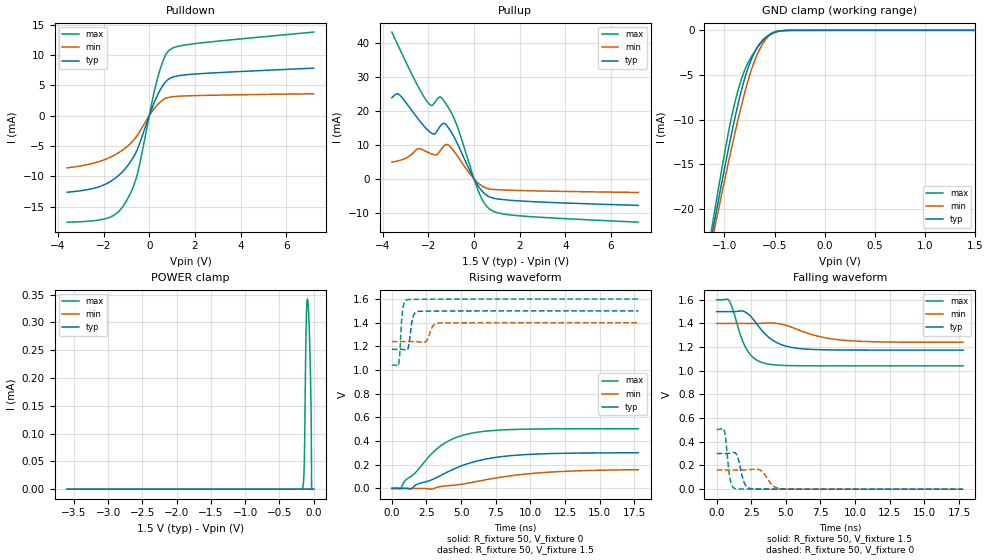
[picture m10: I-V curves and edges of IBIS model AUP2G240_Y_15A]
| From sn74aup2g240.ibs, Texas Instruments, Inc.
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[Model]   AUP2G240_Y_15A
Model_type  3-state
Enable   Active-Low
Vref =   0
Rref =   1E6
Cref =   30p
Vmeas =   0.75
| variable   typ   min   max
C_comp   2.15pF   1.95pF   2.46pF
| C_pullup   2.93pF   2.16pF   3.64pF
| C_pulldown   2.53pF   2.25pF   2.88pF
| C_tri-state   2.15pF   1.95pF   2.46pF
[Temperature Range]   40   100   -40
| Ambient temperature   25   85   -40
[Voltage range]   1.5   1.4   1.6
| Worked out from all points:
|   slope of the pulldown table from 0 to 0.225 V, typ, clamps not added: 101 ohm
|   slope of the pullup table from 0 to 0.225 V, typ, clamps not added: 90.7 ohm
|   GND clamp passes 1 mA (typ) near -0.61 V on its own axis
|   rising waveform, R_fixture 50, V_fixture 0: 20-80 % time 3.92ns typ, 5.36ns min, 2.76ns max; typ from 0 V to 0.301 V
|   falling waveform, R_fixture 50, V_fixture 1.5: 20-80 % time 1.67ns typ, 2.73ns min, 1.07ns max; typ from 1.5 V to 1.18 V
|   rising waveform, R_fixture 50, V_fixture 1.5: 20-80 % time 232ps typ, 317ps min, 180ps max; typ from 1.18 V to 1.5 V
|   falling waveform, R_fixture 50, V_fixture 0: 20-80 % time 381ps typ, 592ps min, 272ps max; typ from 0.302 V to 0 V
[GND Clamp]
| AUP2G240_Y_15A
|   Voltage   I(typ)   I(min)   I(max)
-3.6V     -191.7mA   -177.9mA   -208.5mA
-1.13V    -23.31mA   -24.02mA   -22.49mA
-1.105V   -21.79mA   -22.63mA   -20.79mA
-1.085V   -20.58mA   -21.53mA   -19.44mA
-950mV    -12.76mA   -14.3mA    -10.91mA
-850mV    -7.621mA   -9.344mA   -6.192mA
-785mV    -4.955mA   -6.469mA   -4.124mA
-720mV    -2.969mA   -4.074mA   -2.762mA
-650mV    -1.522mA   -2.167mA   -1.616mA
-580mV    -733.4uA   -902.1uA   -734uA
-390mV    -21.99uA   -24.65uA   -8.299uA
1.5V      139.3pA    22.28nA    27.28pA
[POWER Clamp]
| AUP2G240_Y_15A
|   Voltage   I(typ)   I(min)   I(max)
-3.6V     1.555nA    3.017nA    543.3pA
-170mV    947.8pA    3.23nA     623.5nA
-140mV    6.153nA    7.576nA    33.92uA
-130mV    14.96nA    10.7nA     97.54uA
-110mV    84.92nA    19.18nA    292.2uA
-100mV    170.9nA    22.28nA    332.3uA
-90mV     274.7nA    22.96nA    342.1uA
-70mV     286.4nA    16.34nA    307.8uA
-45mV     32.5nA     4.747nA    195.4uA
-35mV     468.4pA    2.585nA    123.1uA
-30mV     327.7pA    1.919nA    35.79pA
0V        0A         0A         0A
[Pulldown]
| AUP2G240_Y_15A
|   Voltage   I(typ)   I(min)   I(max)
-3.6V     -12.62mA   -8.605mA   -17.56mA
-1.79V    -11.04mA   -6.985mA   -16.83mA
-1.38V    -9.961mA   -6.191mA   -15.93mA
-1.02V    -8.588mA   -5.241mA   -14.16mA
-725mV    -7.016mA   -4.193mA   -11.94mA
-525mV    -5.567mA   -3.252mA   -9.657mA
150mV     1.53mA     832.4uA    2.806mA
420mV     3.835mA    2.043mA    6.955mA
670mV     5.357mA    2.767mA    9.628mA
900mV     6.139mA    3.055mA    10.86mA
1.995V    6.857mA    3.303mA    11.87mA
7.2V      7.827mA    3.609mA    13.77mA
[Pullup]
| AUP2G240_Y_15A
|   Voltage   I(typ)   I(min)   I(max)
-3.6V     23.95mA    4.976mA    43.35mA
-3.25V    24.72mA    5.488mA    38.28mA
-2.46V    17.83mA    8.92mA     27.43mA
-2.06V    14.65mA    7.989mA    22.9mA
-1.74V    13.25mA    7.129mA    22.39mA
-1.475V   15.6mA     8.413mA    24.19mA
-1.17V    15.57mA    10.16mA    21.56mA
-730mV    10.45mA    6.821mA    15.42mA
200mV     -2.247mA   -1.333mA   -3.769mA
690mV     -5.334mA   -2.972mA   -8.934mA
1.94V     -6.46mA    -3.399mA   -10.85mA
7.2V      -7.803mA   -3.988mA   -12.76mA
[Ramp]
| AUP2G240_Y_15A
| variable   typ   min   max
dV/dt_r   0.18/4.02E-09   0.10/5.61E-09   0.30/2.79E-09
dV/dt_f   0.20/1.69E-09   0.10/2.76E-09   0.34/1.08E-09
R_load = 50
[Rising Waveform]
| AUP2G240_Y_15A
R_fixture =   50
C_fixture =   0
L_fixture =   0
V_fixture =   0
V_fixture_min = 0
V_fixture_max = 0
|   Time   V(typ)   V(min)   V(max)
0s        6.328nV    24.54nV    515.8pV
649ps     19.85uV    -7.754uV   -1.988mV
929ps     559.1uV    -16.46uV   61.15mV
1.373ns   -5.623mV   -821.6nV   101.1mV
1.821ns   34.84mV    278.7uV    147.9mV
2.849ns   71.57mV    -6.275mV   290.2mV
3.593ns   113.2mV    16.93mV    365.3mV
5.421ns   206.9mV    43.05mV    457.9mV
9.509ns   284.9mV    119.6mV    500.4mV
17.8ns    301.2mV    158.3mV    504.4mV
[Falling Waveform]
| AUP2G240_Y_15A
R_fixture =   50
C_fixture =   0
L_fixture =   0
V_fixture =   1.5
V_fixture_min = 1.4
V_fixture_max = 1.6
|   Time   V(typ)   V(min)   V(max)
0s        1.5V       1.4V       1.6V
897ps     1.5V       1.4V       1.593V
1.753ns   1.506V     1.4V       1.293V
2.117ns   1.493V     1.4V       1.193V
2.661ns   1.433V     1.4V       1.111V
3.421ns   1.321V     1.402V     1.065V
4.649ns   1.222V     1.394V     1.046V
6.297ns   1.185V     1.329V     1.042V
9.705ns   1.175V     1.253V     1.042V
17.8ns    1.175V     1.241V     1.042V
[Rising Waveform]
| AUP2G240_Y_15A
R_fixture =   50
C_fixture =   0
L_fixture =   0
V_fixture =   1.5
V_fixture_min = 1.4
V_fixture_max = 1.6
|   Time   V(typ)   V(min)   V(max)
0s        1.175V     1.24V      1.042V
473ps     1.175V     1.24V      1.042V
561ps     1.175V     1.24V      1.119V
793ps     1.175V     1.24V      1.518V
1.137ns   1.174V     1.241V     1.595V
1.517ns   1.444V     1.241V     1.597V
1.885ns   1.495V     1.239V     1.598V
2.453ns   1.498V     1.24V      1.599V
3.389ns   1.499V     1.397V     1.599V
17.8ns    1.5V       1.4V       1.6V
[Falling Waveform]
| AUP2G240_Y_15A
R_fixture =   50
C_fixture =   0
L_fixture =   0
V_fixture =   0
V_fixture_min = 0
V_fixture_max = 0
|   Time   V(typ)   V(min)   V(max)
0s        301.6mV    161.8mV    504.4mV
549ps     301.2mV    161.8mV    499.6mV
989ps     305.1mV    161.6mV    76.74mV
1.385ns   302.5mV    161.5mV    4.083mV
2.001ns   53.38mV    162.5mV    586.7uV
2.477ns   5.083mV    166.2mV    224.3uV
3.201ns   1.087mV    157.7mV    70uV
4.021ns   336.3uV    33.67mV    20.67uV
4.613ns   171uV      4.394mV    8.695uV
17.8ns    53.46nV    767.4nV    16.45nV
